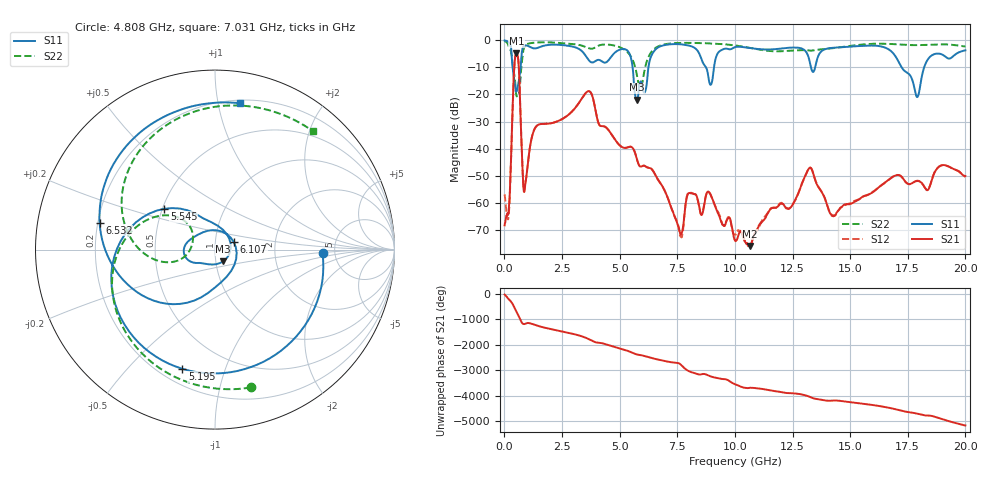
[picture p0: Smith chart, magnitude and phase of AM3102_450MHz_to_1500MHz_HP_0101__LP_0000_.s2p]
!Agilent Technologies,E8364B,MY43040894,A.07.50.67
!Agilent E8364B: A.07.50.67
!Date: Thursday, January 11, 2018 05:39:22
!Correction: S11(Full 2 Port(1,2))
!S21(Full 2 Port(1,2))
!S12(Full 2 Port(1,2))
!S22(Full 2 Port(1,2))
!S2P File: Measurements: S11, S21, S12, S22:
# Hz S  dB  R 50
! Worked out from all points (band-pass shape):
!   1601 points, 10 MHz to 20 GHz, reference 50 ohm
!   highest |S21| = -4.79 dB at 522.2 MHz (marker M1); lowest = -76.0 dB at 10.64 GHz (marker M2)
!   |S21| within 3 dB of the highest: 448.9 MHz to 609 MHz (160 MHz wide, 30.3 % of centre)
!   lowest |S11| = -22.0 dB at 5.745 GHz (marker M3), VSWR 1.17, Z = 54.4 - j7.11 ohm
!   |S11| at or under -10 dB: 357.4 MHz to 703.2 MHz (345.8 MHz wide, 65.2 % of centre); 5.563 GHz to 6.249 GHz (685.5 MHz wide, 11.6 % of centre); 17.24 GHz to 18.21 GHz (974.1 MHz wide, 5.5 % of centre)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
!   |S22| runs from -20.7 to -0.3 dB; largest |S21 - S12| = 0.003
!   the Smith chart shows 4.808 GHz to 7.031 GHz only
!   S11 on the Smith chart (normalised r, x): 4.808 GHz: 3.98, -0.26; 5.195 GHz: 0.29, -0.72; 5.545 GHz: 0.51, +0.27; 6.107 GHz: 1.23, +0.10; 6.532 GHz: 0.21, +0.11; 7.031 GHz: 0.22, +1.16
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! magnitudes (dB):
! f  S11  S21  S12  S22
! 10 MHz  -0.1  -68.4  -56.9  -0.3
! 197.4 MHz  -0.7  -61.7  -63.7  -2.5
! 522.2 MHz  -18.8  -4.8  -4.8  -20.5
! 884.6 MHz  -1.9  -54.7  -54.6  -2.1
! 1.359 GHz  -3.0  -32.0  -32.0  -0.8
! 3.346 GHz  -3.9  -21.7  -21.7  -1.9
! 4.808 GHz  -4.4  -36.8  -36.8  -2.0
! 5.195 GHz  -3.2  -39.7  -39.7  -3.4
! 5.545 GHz  -8.8  -39.6  -39.6  -6.9
! 5.745 GHz  -22.0  -43.8  -43.7  -12.6
! 6.107 GHz  -18.9  -46.5  -46.5  -10.0
! 6.532 GHz  -3.6  -49.4  -49.5  -3.0
! 6.682 GHz  -2.6  -51.7  -51.7  -2.2
! 7.031 GHz  -1.6  -57.0  -57.0  -1.4
! 8.943 GHz  -16.5  -57.0  -57.0  -1.1
! 10.01 GHz  -2.5  -74.0  -71.8  -1.9
! 10.64 GHz  -2.8  -76.0  -75.7  -2.8
! 13.34 GHz  -11.1  -47.7  -47.7  -3.8
! 14.27 GHz  -2.8  -65.0  -64.8  -2.9
! 16.68 GHz  -3.4  -51.5  -51.5  -1.3
! 17.9 GHz  -20.9  -52.0  -51.9  -1.8
! 20 GHz  -3.7  -50.1  -50.4  -2.3
